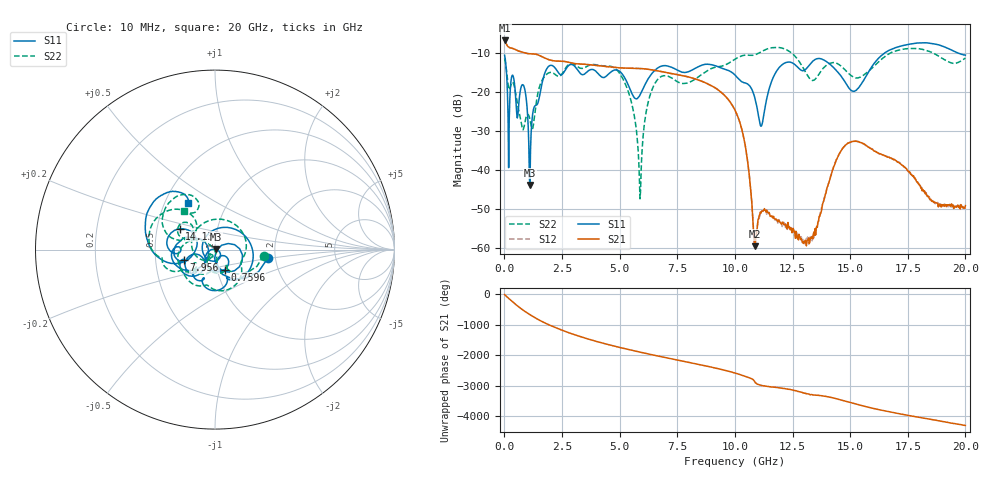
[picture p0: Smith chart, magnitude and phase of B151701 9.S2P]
!  2-Port S-parameters saved by WinCal
! VAR MeasName=S-Parameters (CALIBRATED_DATA) read from VNA (N5244A)
! VAR MeasDate=2015-12-24 19:09:07
! VAR NAME=B151701 9
! VAR FILENAME=B151701 9.S2P
! VAR DATE=2015-12-24 19:09:07
! VAR PHYS_PORTS=1,3
# Hz S DB R 50
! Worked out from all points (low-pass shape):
!   801 points, 10 MHz to 20 GHz, reference 50 ohm
!   highest |S21| = -6.66 dB at 10 MHz (marker M1); lowest = -59.6 dB at 10.88 GHz (marker M2)
!   |S21| within 3 dB of the highest: start of sweep to 773.2 MHz
!   lowest |S11| = -43.9 dB at 1.109 GHz (marker M3), VSWR 1.01, Z = 50.6 + j0.142 ohm
!   |S11| at or under -10 dB: start of sweep to 16.47 GHz; 19.72 GHz to end of sweep
!   |S22| runs from -47.4 to -8.4 dB; largest |S21 - S12| = 0.0012
!   S11 on the Smith chart (normalised r, x): 10 MHz: 1.83, -0.18; 759.6 MHz: 1.09, -0.25; 7.956 GHz: 0.70, -0.09; 14.13 GHz: 0.66, +0.16; 20 GHz: 0.65, +0.37
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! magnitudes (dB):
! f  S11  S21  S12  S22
! 10 MHz  -10.5  -6.7  -6.7  -11.3
! 184.9 MHz  -39.4  -8.3  -8.3  -18.7
! 759.6 MHz  -18.2  -9.6  -9.6  -28.8
! 1.109 GHz  -43.9  -10.1  -10.1  -27.0
! 1.884 GHz  -13.5  -11.5  -11.5  -15.1
! 3.358 GHz  -15.4  -12.8  -12.7  -13.9
! 5.082 GHz  -15.1  -13.7  -13.7  -15.9
! 5.582 GHz  -20.9  -13.8  -13.8  -24.4
! 5.882 GHz  -20.7  -13.9  -13.9  -47.4
! 6.207 GHz  -16.8  -14.1  -14.0  -23.4
! 6.682 GHz  -13.6  -14.5  -14.5  -16.5
! 7.956 GHz  -14.7  -16.0  -16.0  -17.6
! 10.01 GHz  -15.6  -24.6  -24.6  -11.5
! 10.48 GHz  -17.7  -34.8  -34.9  -10.4
! 10.88 GHz  -21.8  -59.6  -59.3  -10.3
! 11.15 GHz  -28.6  -50.7  -50.7  -9.5
! 11.93 GHz  -13.6  -53.1  -53.0  -8.5
! 13.35 GHz  -12.1  -57.1  -58.2  -16.9
! 14.13 GHz  -12.8  -42.3  -42.3  -12.5
! 15.18 GHz  -19.8  -32.6  -32.7  -16.2
! 16.68 GHz  -9.2  -36.7  -36.6  -10.1
! 20 GHz  -10.4  -49.2  -49.9  -11.2
